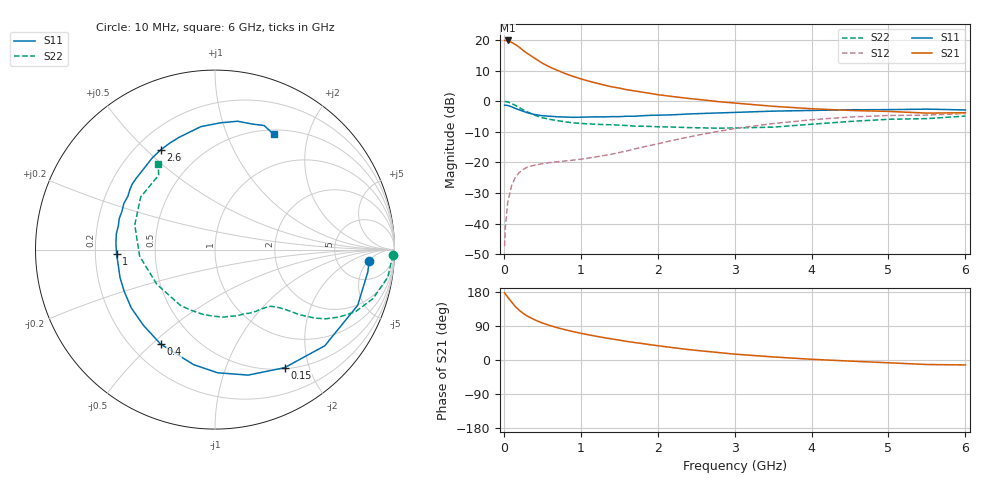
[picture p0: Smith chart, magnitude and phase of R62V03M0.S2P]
! SIEMENS Small Signal Semiconductors
! BFR193
! Si NPN RF Bipolar Junction Transistor in SOT23
! VCE = 2 V  IC = 3 mA
! Common Emitter S-Parameters:  May  1996
# GHz  S  MA  R  50
!  f  S11  S21  S12  S22
! GHz  MAG  ANG  MAG  ANG  MAG  ANG  MAG  ANG
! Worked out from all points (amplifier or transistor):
!   36 points, 10 MHz to 6 GHz, reference 50 ohm
!   highest |S21| = 19.9 dB at 50 MHz (marker M1)
!   |S21| within 3 dB of that: start of sweep to 238.6 MHz
!   unconditionally stable (mu >= 1): 1.033 GHz to 2.056 GHz
!   at 250 MHz: K = 0.30, MSG = 19.5 dB, |S12| = -22.3 dB
!   at 1.4 GHz: K = 1.10, MAG = 9.1 dB, |S12| = -17.3 dB
!   at 6 GHz: K = 0.99, MSG = 0.1 dB, |S12| = -4.0 dB
!   S11 on the Smith chart (normalised r, x): 10 MHz: 11, -5; 150 MHz: 0.52, -1.63; 400 MHz: 0.32, -0.53; 1 GHz: 0.29, -0.02; 2.6 GHz: 0.30, +0.55; 6 GHz: 0.56, +1.48
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0.01  0.8615 -4.3  9.805 177.5  0.0043 88.9  0.9946 -1.8
0.02  0.8603 -8.4  9.819 174.3  0.0089 86.1  0.9857 -3.6
0.05  0.8535 -21.3  9.829 166.0  0.0221 78.8  0.9749 -9.1
0.1  0.8132 -41.2  9.181 153.2  0.0417 69.0  0.922 -17.2
0.15  0.7637 -59.5  8.425 140.8  0.0574 60.3  0.8563 -23.8
0.2  0.7232 -75.2  7.647 131.4  0.0684 54.2  0.7875 -28.5
0.25  0.6864 -88.8  6.767 123.3  0.0768 49.0  0.7259 -32.1
0.3  0.6521 -100.5  6.099 116.5  0.0835 45.6  0.6758 -34.4
0.4  0.6074 -119.9  5.048 106.2  0.0906 41.2  0.5922 -37.7
0.5  0.5803 -133.6  4.187 97.7  0.0954 39.2  0.5376 -39.5
0.6  0.5684 -145.1  3.604 90.9  0.0997 38.3  0.5058 -40.8
0.8  0.5518 -163.4  2.823 79.7  0.1061 40.0  0.4615 -43.7
1  0.549 -177.4  2.319 70.6  0.113 44.1  0.4344 -47.2
1.1  0.553 176.5  2.137 66.5  0.1181 46.5  0.4267 -49.5
1.3  0.5546 166.2  1.842 59.1  0.1298 50.5  0.4155 -53.9
1.6  0.5693 153.1  1.541 49.0  0.1546 55.8  0.4013 -62.3
2.2  0.6008 131.2  1.191 32.5  0.2302 58.9  0.3788 -83.0
2.6  0.6326 118.6  1.047 23.4  0.2916 56.1  0.3669 -100.7
3.5  0.6895 96.6  0.827 8.1  0.4322 42.0  0.3775 -149.2
4.5  0.7262 80.0  0.708 -2.9  0.5521 23.1  0.4677 162.9
5.5  0.7435 68.4  0.64 -11.9  0.5942 5.0  0.5202 127.1
6  0.7203 63.0  0.65 -13.0  0.6287 -0.1  0.5727 123.5
